|Texas Instruments Incorporated
| Dual 16-Bit,250 MSPS Analog-Digital converters
| Marketing part#   Digital Voltage Range   Package-type   #pins
| ADS42JB69   1.8V-3.6V   QFN   64
[IBIS Ver]   4.1
[File name]   ads42jb69.ibs
[File Rev]   1.1
[Date]   6/12/2013
[Source]
| Texas Instruments Incorporated.
| Analog-eLab Design Center, HPA
| 12500 TI Blvd
| Dallas, TX -75243
[Notes]   Revision History:
| Rev 1.1: 6/12/2012
| - Differential IBIS files are generated with Rref=50ohms,Vref=VDD
| - V-T Tables are generated with V_fix=VDD(1.8-Typ,1.7-Min,1.9-Max).
| Rev 1.0: 5/24/2013
| - Initial version of the model
| - Model generated from simulations in TISPICE
| - Model matched to SPICE simulation
| - C_comp although listed in numerical order of value are
|   obtained from varying PVT conditions. For PVT conditions for
|   each specific value refer the buffer description under
|   respective [Model]. IBIS model user is responsible for using
|   appropriate C_comp to simulate for Signal Integrity.
[Disclaimer]
| This model is designed as an aid for customers of Texas Instruments.
| TI and its licensors and suppliers make no warranties, either expressed
| or implied, with respect to this  model, including the warranties of
| merchantability or fitness for a particular purpose. The model is
| provided solely on an "as is" basis. The entire risk as to its quality
| and performance is with the customer.
|*  EXCEPTION:   *
|*  - For model reset ,there will be a leakage in the Power clamp I-V   *
|*   due to pullup resistor R1(RES3T_NPL_SIBLK) connected to the pad   *
|*  - For model sclk, there will be a leakage in the power clamp  I-V table *
|*   due to the resistor R1(RES3T_NPL_SIBLK) connected to the pad   *
|*  - For model sen, there will be a leakage in the ground clamp I-V table  *
|*   due to the R1(RES3T_NPL_SIBLK) connected to the pad   *
|*  - For model sync_sysref, there will be a leakage current in the power   *
|*   and ground clamp I-V Table due to the series resistor(RES3T_NPL_SIBLK)*
|*   connected between SYNCP and SYNCM   *
|*  - For model clk_diff, there will be a leakage current in the power and  *
|*   ground clamp I-V Table due to the series resistor   *
|*   (RES3T_NPL_SIBLK) connected between CLKINP and CLKINM   *
|*   connected to pad.   *
|*  - For model diff_out_mode*,[Pulldown] curve does not pass through a   *
|*   zero/zero due to the leakage current by transistors MN_INP and MN_INM *
|*   (NCH4T_1P8V) connected to pad.
[Copyright]
(C) Copyright 2013 Texas Instruments Incorporated.All rights reserved.
|   ADS42JB69
[Component]   ADS42JB69
[Manufacturer]   TI
[Package]   |64 QFN   -  RGC package
|   typ   min   max
R_pkg   0.34176   0.15316   0.41243
L_pkg   1.83875nH   1.20045nH   2.21079nH
C_pkg   0.23608pF   0.21142pF   0.27033pF
[Pin]  signal_name   model_name   R_pin   L_pin   C_pin
1   DGND   gnd   0.00508   0.07972nH  2.75774pF
2   DRVDD   power   0.20289   1.72532nH  0.31771pF
3   DGND   gnd   0.39610   2.11609nH  0.24588pF
4   MODE   gnd   0.39706   2.12166nH  0.24904pF
5   STBY   sclk   0.39157   2.08965nH  0.24801pF
6   PDN_GBL   sclk   0.38637   2.05925nH  0.24643pF
7   DRVDD   power   0.19240   1.60777nH  0.31097pF
8   SYNCP   sync_sysref   0.36747   1.94925nH  0.23907pF
9   SYNCM   sync_sysref   0.35294   1.86535nH  0.22375pF
10   CTRL2   sclk   0.36517   1.93585nH  0.23185pF
11   AVDD   power   0.17669   1.43363nH  0.29430pF
12   AGND   gnd   0.17559   1.42103nH  0.29778pF
13   INBP   nc   0.17868   1.45403nH  0.30209pF
14   INBM   nc   0.18571   1.53067nH  0.31181pF
15   AGND   gnd   0.19624   1.64683nH  0.32492pF
16   AVDD   power   0.20977   1.83438nH  0.30309pF
17   AVDD3V   power   0.20807   1.87499nH  0.29105pF
18   AVDD   power   0.19663   1.68553nH  0.31155pF
19   AGND   gnd   0.35883   1.90489nH  0.23545pF
20   AGND   gnd   0.16840   1.38113nH  0.26874pF
21   VCM   power   0.16680   1.35141nH  0.27550pF
22   AVDD   power   0.16552   1.33736nH  0.28405pF
23   AGND   gnd   0.15741   1.24818nH  0.27631pF
24   CLKINM   clk_diff   0.15317   1.20151nH  0.27033pF
25   CLKINP   clk_diff   0.15316   1.20045nH  0.27032pF
26   AGND   gnd   0.15739   1.24512nH  0.27616pF
27   AVDD   power   0.16549   1.33228nH  0.28030pF
28   AGND   gnd   0.32874   1.72925nH  0.21694pF
29   SYSREFP   sync_sysref   0.34930   1.84926nH  0.22981pF
30   SYSREFM   sync_sysref   0.38610   2.06439nH  0.25017pF
31   AVDD   power   0.19663   1.67698nH  0.32263pF
32   AVDD3V   power   0.20807   1.85722nH  0.30055pF
33   AVDD   power   0.20977   1.85169nH  0.30300pF
34   AGND   gnd   0.19624   1.65348nH  0.32499pF
35   INAM   nc   0.18571   1.53540nH  0.31183pF
36   INAP   nc   0.17868   1.45670nH  0.30207pF
37   AGND   gnd   0.17559   1.42159nH  0.29766pF
38   AVDD   power   0.17669   1.43203nH  0.29318pF
39   CTRL1   sclk   0.36517   1.93585nH  0.22779pF
40   AVDD   power   0.17652   1.43030nH  0.27031pF
41   SEN   sen   0.35702   1.88875nH  0.23326pF
42   SDATA   sclk   0.35953   1.90325nH  0.23004pF
43   SCLK   sclk   0.36241   1.91995nH  0.23484pF
44   RESET   reset   0.36567   1.93886nH  0.23277pF
45   SDOUT   sdout   0.36929   1.95986nH  0.23789pF
46   DGND   gnd   0.39610   2.11609nH  0.24430pF
47   DRVDD   power   0.20289   1.71779nH  0.31755pF
48   DGND   gnd   0.41527   2.23108nH  0.23261pF
49   DRVDD   power   0.20750   1.88200nH  0.28965pF
50   DGND   gnd   0.37587   1.99616nH  0.23859pF
51   DA1M   diff_out_mode   0.41243   2.21079nH  0.26286pF
52   DA1P   diff_out_mode   0.37014   1.96236nH  0.24054pF
53   DA0M   diff_out_mode   0.34837   1.83455nH  0.22938pF
54   DA0P   diff_out_mode   0.32080   1.67315nH  0.21861pF
55   IOVDD   power   0.15490   1.22609nH  0.27313pF
56   DB0P   diff_out_mode   0.30475   1.57925nH  0.21161pF
57   DB0M   diff_out_mode   0.31135   1.61785nH  0.21142pF
58   DB1P   diff_out_mode   0.32251   1.68315nH  0.21675pF
59   DB1M   diff_out_mode   0.35096   1.84985nH  0.23287pF
60   DRVDD   power   0.17698   1.46512nH  0.29116pF
61   OVRA   over_range   0.35602   1.87946nH  0.23599pF
62   OVRB   over_range   0.36237   1.91679nH  0.23566pF
63   DGND   gnd   0.37707   2.00318nH  0.24097pF
64   DRVDD   power   0.20820   1.89078nH  0.28990pF
[Diff_pin]   inv_pin   vdiff   tdelay_typ   tdelay_min   tdelay_max
8   9   NA   NA   NA   NA
25   24   NA   NA   NA   NA
29   30   NA   NA   NA   NA
52   51   0.4   NA   NA   NA
54   53   0.4   NA   NA   NA
56   57   0.4   NA   NA   NA
58   59   0.4   NA   NA   NA
[Model Selector] diff_out_mode
diff_out_mode0_p 1.8V Differential output with currsel <3:0> set to 0000, 16mA
diff_out_mode0_n 1.8V Differential output with currsel <3:0> set to 0000, 16mA
diff_out_mode1_p 1.8V Differential output with currsel <3:0> set to 0001, 15mA
diff_out_mode1_n 1.8V Differential output with currsel <3:0> set to 0001, 15mA
diff_out_mode2_p 1.8V Differential output with currsel <3:0> set to 0010, 14mA
diff_out_mode2_n 1.8V Differential output with currsel <3:0> set to 0010, 14mA
diff_out_mode3_p 1.8V Differential output with currsel <3:0> set to 0011, 13mA
diff_out_mode3_n 1.8V Differential output with currsel <3:0> set to 0011, 13mA
diff_out_mode4_p 1.8V Differential output with currsel <3:0> set to 0100, 20mA
diff_out_mode4_n 1.8V Differential output with currsel <3:0> set to 0100, 20mA
diff_out_mode5_p 1.8V Differential output with currsel <3:0> set to 0101, 19mA
diff_out_mode5_n 1.8V Differential output with currsel <3:0> set to 0101, 19mA
diff_out_mode6_p 1.8V Differential output with currsel <3:0> set to 0110, 18mA
diff_out_mode6_n 1.8V Differential output with currsel <3:0> set to 0110, 18mA
diff_out_mode7_p 1.8V Differential output with currsel <3:0> set to 0111, 17mA
diff_out_mode7_n 1.8V Differential output with currsel <3:0> set to 0111, 17mA
diff_out_mode8_p 1.8V Differential output with currsel <3:0> set to 1000, 8mA
diff_out_mode8_n 1.8V Differential output with currsel <3:0> set to 1000, 8mA
diff_out_mode9_p 1.8V Differential output with currsel <3:0> set to 1001, 7mA
diff_out_mode9_n 1.8V Differential output with currsel <3:0> set to 1001, 7mA
diff_out_mode10_p 1.8V Differential output with currsel <3:0> set to 1010, 6mA
diff_out_mode10_n 1.8V Differential output with currsel <3:0> set to 1010, 6mA
diff_out_mode11_p 1.8V Differential output with currsel <3:0> set to 1011, 5mA
diff_out_mode11_n 1.8V Differential output with currsel <3:0> set to 1011, 5mA
diff_out_mode12_p 1.8V Differential output with currsel <3:0> set to 1100, 12mA
diff_out_mode12_n 1.8V Differential output with currsel <3:0> set to 1100, 12mA
diff_out_mode13_p 1.8V Differential output with currsel <3:0> set to 1101, 11mA
diff_out_mode13_n 1.8V Differential output with currsel <3:0> set to 1101, 11mA
diff_out_mode14_p 1.8V Differential output with currsel <3:0> set to 1110, 10mA
diff_out_mode14_n 1.8V Differential output with currsel <3:0> set to 1110, 10mA
diff_out_mode15_p 1.8V Differential output with currsel <3:0> set to 1111, 9mA
diff_out_mode15_n 1.8V Differential output with currsel <3:0> set to 1111, 9mA
[Model Selector]sync_sysref
sync_sysref_p   1.8V Differential input
sync_sysref_n   1.8V Differential input
[Model Selector]  clk_diff
clk_diff_p   3.3V Differential input
clk_diff_n   3.3V Differential input
| Models and submodels in the file (41): reset (Input), sclk (Input), sen (Input), over_range (Output), sdout (Output), sync_sysref_p (Input), sync_sysref_n (Input), clk_diff_p (Input), clk_diff_n (Input), diff_out_mode0_p (Output), diff_out_mode0_n (Output), diff_out_mode1_p (Output), diff_out_mode1_n (Output), diff_out_mode2_p (Output), diff_out_mode2_n (Output), diff_out_mode3_p (Output), diff_out_mode3_n (Output), diff_out_mode4_p (Output), diff_out_mode4_n (Output), diff_out_mode5_p (Output), diff_out_mode5_n (Output), diff_out_mode6_p (Output), diff_out_mode6_n (Output), diff_out_mode7_p (Output), diff_out_mode7_n (Output), diff_out_mode8_p (Output), diff_out_mode8_n (Output), diff_out_mode9_p (Output), diff_out_mode9_n (Output), diff_out_mode10_p (Output), diff_out_mode10_n (Output), diff_out_mode11_p (Output), diff_out_mode11_n (Output), diff_out_mode12_p (Output), diff_out_mode12_n (Output), diff_out_mode13_p (Output), diff_out_mode13_n (Output), diff_out_mode14_p (Output), diff_out_mode14_n (Output), diff_out_mode15_p (Output), diff_out_mode15_n (Output)
